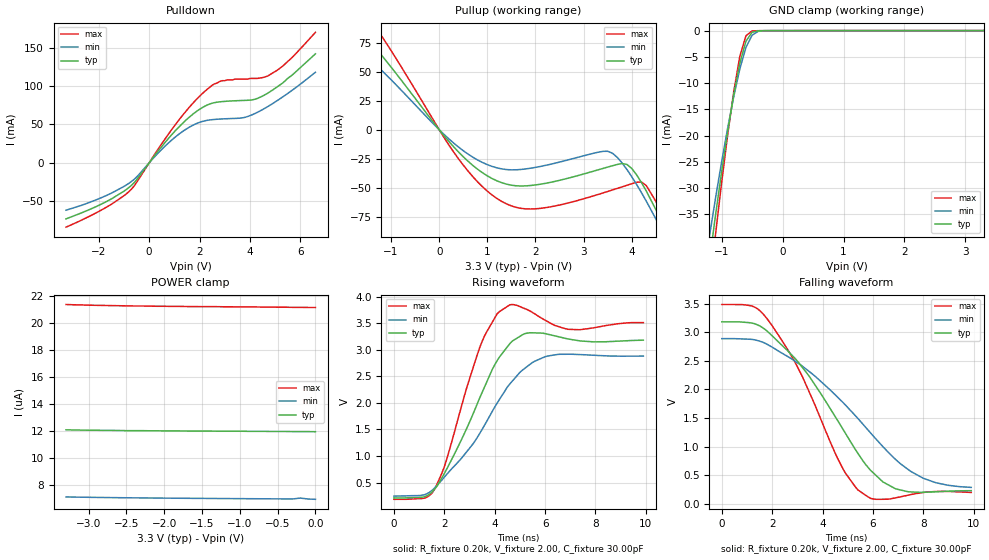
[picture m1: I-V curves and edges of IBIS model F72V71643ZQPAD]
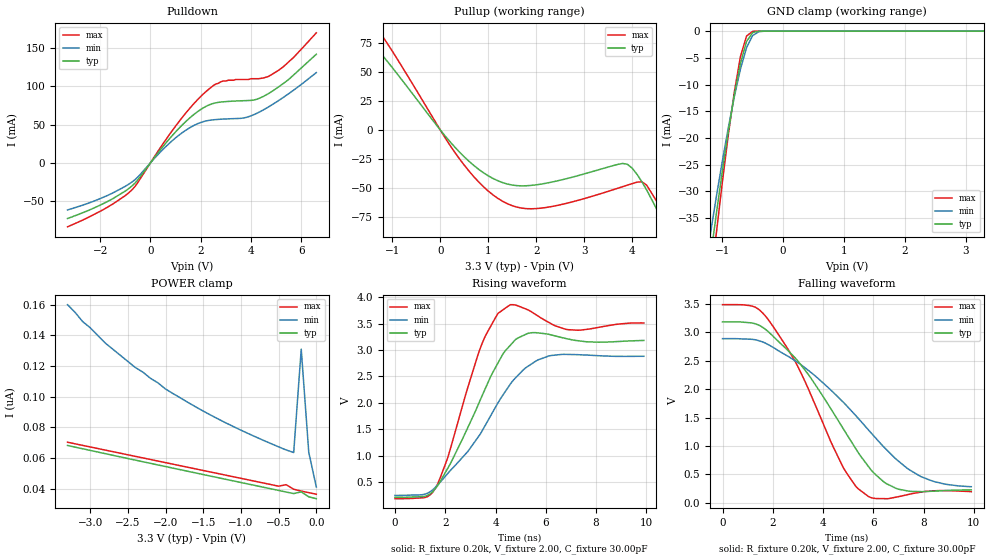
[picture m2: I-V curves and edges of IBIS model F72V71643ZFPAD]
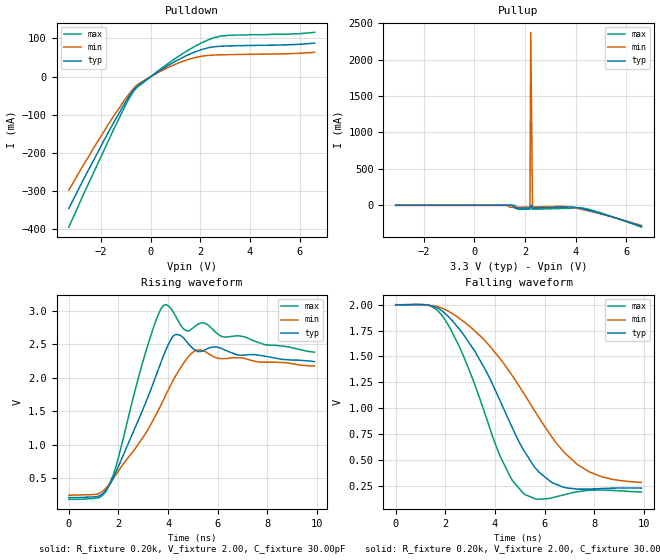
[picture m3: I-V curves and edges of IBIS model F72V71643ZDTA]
| IBIS file f72v7164.ibs created by s2ibis2 version 1.1
| North Carolina State University Electronics Research Laboratory  1995
[IBIS ver]   2.1
[File name]   f72v7164.ibs
[File Rev]   1.0
[Date]   09/11/2000
[Source]   Integrated Device Technology, Inc.
[Notes]   1. Temperatures: typ=25C, min=85C, max=-40C 2. Cemos9_3v
   process. 3. Ramp rates based on 50 ohm load.
[Copyright]   Copyright 1999, Integrated Device Technology, Inc.
|   Component idt72v71643z
[Component]   idt72v71643z
[Manufacturer]   Integrated Device Technology
[Package]
| variable   typ   min   max
R_pkg   0.75   0.60   0.90
L_pkg   8.10nH   8.30nH   9.90nH
C_pkg   0.53pF   0.46pF   0.60pF
[Pin]  signal_name   model_name   R_pin   L_pin   C_pin
1   ODE   F72V71643ZTTL
2   RESET   F72V71643ZTTL
3   GND   GND
4   CLK   F72V71643ZTTL
5   FOI   F72V71643ZTTL
6   FE_HCLK   F72V71643ZTTL
7   WFPS   F72V71643ZTTL
8   VCC   POWER
9   TMS   F72V71643ZTTLPU
10   TDI   F72V71643ZTTLPU
11   TDO   F72V71643ZFPAD
12   TCK   F72V71643ZTTL
13   TRST   F72V71643ZTTLPU
14   GND   GND
15   DS   F72V71643ZTTL
16   CS   F72V71643ZTTL
17   R_W   F72V71643ZTTL
18   VCC   POWER
19   A0   F72V71643ZTTL
20   A1   F72V71643ZTTL
21   A2   F72V71643ZTTL
22   A3   F72V71643ZTTL
23   A4   F72V71643ZTTL
24   A5   F72V71643ZTTL
25   GND   GND
26   A6   F72V71643ZTTL
27   A7   F72V71643ZTTL
28   A8   F72V71643ZTTL
29   A9   F72V71643ZTTL
30   A10   F72V71643ZTTL
31   A11   F72V71643ZTTL
32   A12   F72V71643ZTTL
33   A13   F72V71643ZTTL
34   A14   F72V71643ZTTL
35   DTA   F72V71643ZDTA
36   VCC   POWER
37   D15   F72V71643ZQPAD
38   D14   F72V71643ZQPAD
39   GND   GND
40   D13   F72V71643ZQPAD
41   D12   F72V71643ZQPAD
42   VCC   POWER
43   D11   F72V71643ZQPAD
44   D10   F72V71643ZQPAD
45   GND   GND
46   D9   F72V71643ZQPAD
47   D8   F72V71643ZQPAD
48   VCC   POWER
49   D7   F72V71643ZQPAD
50   D6   F72V71643ZQPAD
51   GND   GND
52   D5   F72V71643ZQPAD
53   D4   F72V71643ZQPAD
54   VCC   POWER
55   D3   F72V71643ZQPAD
56   D2   F72V71643ZQPAD
57   GND   GND
58   D1   F72V71643ZQPAD
59   D0   F72V71643ZQPAD
60   VCC   POWER
61   TX31   F72V71643ZFPAD
62   TX30   F72V71643ZFPAD
63   GND   GND
64   TX29   F72V71643ZFPAD
65   TX28   F72V71643ZFPAD
66   VCC   POWER
67   TX27   F72V71643ZFPAD
68   TX26   F72V71643ZFPAD
69   GND   GND
70   TX25   F72V71643ZFPAD
71   TX24   F72V71643ZFPAD
72   VCC   POWER
73   RX31   F72V71643ZTTL
74   RX30   F72V71643ZTTL
75   Rx29   F72V71643ZTTL
76   RX28   F72V71643ZTTL
77   RX27   F72V71643ZTTL
78   RX26   F72V71643ZTTL
79   RX25   F72V71643ZTTL
80   RX24   F72V71643ZTTL
81   GND   GND
82   TX23   F72V71643ZFPAD
83   TX22   F72V71643ZFPAD
84   VCC   POWER
85   TX21   F72V71643ZFPAD
86   TX20   F72V71643ZFPAD
87   GND   GND
88   TX19   F72V71643ZFPAD
89   TX18   F72V71643ZFPAD
90   VCC   POWER
91   TX17   F72V71643ZFPAD
92   TX16   F72V71643ZFPAD
93   GND   GND
94   RX23   F72V71643ZTTL
95   RX22   F72V71643ZTTL
96   RX21   F72V71643ZTTL
97   RX20   F72V71643ZTTL
98   RX19   F72V71643ZTTL
99   RX18   F72V71643ZTTL
100   RX17   F72V71643ZTTL
101   RX16   F72V71643ZTTL
102   VCC   POWER
103   TX15   F72V71643ZFPAD
104   TX14   F72V71643ZFPAD
105   GND   GND
106   TX13   F72V71643ZFPAD
107   TX12   F72V71643ZFPAD
108   VCC   POWER
109   TX11   F72V71643ZFPAD
110   TX10   F72V71643ZFPAD
111   GND   GND
112   TX9   F72V71643ZFPAD
113   TX8   F72V71643ZFPAD
114   VCC   POWER
115   RX15   F72V71643ZTTL
116   RX14   F72V71643ZTTL
117   RX13   F72V71643ZTTL
118   RX12   F72V71643ZTTL
119   RX11   F72V71643ZTTL
120   RX10   F72V71643ZTTL
121   RX9   F72V71643ZTTL
122   RX8   F72V71643ZTTL
123   GND   GND
124   TX7   F72V71643ZFPAD
125   TX6   F72V71643ZFPAD
126   VCC   POWER
127   TX5   F72V71643ZFPAD
128   TX4   F72V71643ZFPAD
129   GND   GND
130   TX3   F72V71643ZFPAD
131   TX2   F72V71643ZFPAD
132   VCC   POWER
133   TX1   F72V71643ZFPAD
134   TX0   F72V71643ZFPAD
135   GND   GND
136   RX7   F72V71643ZTTL
137   RX6   F72V71643ZTTL
138   RX5   F72V71643ZTTL
139   RX4   F72V71643ZTTL
140   RX3   F72V71643ZTTL
141   RX2   F72V71643ZTTL
142   RX1   F72V71643ZTTL
143   RX0   F72V71643ZTTL
144   VCC   POWER
| Models and submodels in the file (5): F72V71643ZQPAD (I/O), F72V71643ZFPAD (3-state), F72V71643ZDTA (Output), F72V71643ZTTL (Input), F72V71643ZTTLPU (Input)
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| FIN  FIN   dummy_model
| FOEL FOEL   dummy_model
| QIN  QIN   dummy_model
| QOEL QOEL   dummy_model
| DIN  DIN   dummy_model
|   Model F72V71643ZQPAD
[Model]   F72V71643ZQPAD
Model_type   I/O
Polarity   Non-Inverting
Enable   Active-Low
Vinl =  0.000V
Vinh =  3.000V
Vmeas =  1.500V
C_comp   3.00pF   NA   NA
[Temperature Range]   25.00   85.00   -40.00
[Voltage Range]   3.30V   3.00V   3.60V
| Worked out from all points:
|   slope of the pulldown table from 0 to 0.495 V, typ, clamps not added: 23.4 ohm
|   slope of the pullup table from 0 to 0.495 V, typ, clamps not added: 21.5 ohm
|   GND clamp passes 1 mA (typ) near -0.54 V on its own axis
|   rising waveform, R_fixture 0.20k, V_fixture 2.00, C_fixture 30.00pF: 20-80 % time 1.71ns typ, 2.27ns min, 1.23ns max; typ from 0.211 V to 3.18 V
|   falling waveform, R_fixture 0.20k, V_fixture 2.00, C_fixture 30.00pF: 20-80 % time 2.7ns typ, 3.51ns min, 2.11ns max; typ from 3.18 V to 0.229 V
[Pulldown]
| voltage   I(typ)   I(min)   I(max)
-3.3V     -72.9mA    -61.6mA    -83.7mA
-1.7V     -50.47mA   -42.52mA   -57.8mA
-800mV    -32mA      -26.54mA   -37.34mA
1.2V      47.36mA    37.84mA    56.62mA
1.9V      67.48mA    51.48mA    83.43mA
2.5V      77.68mA    56.27mA    101mA
2.9V      79.82mA    57.23mA    107mA
3.8V      81.37mA    59.31mA    109mA
4.2V      82.87mA    64.29mA    110mA
4.7V      90.61mA    73.16mA    113mA
5.3V      104mA      85.84mA    126mA
6.6V      142mA      118mA      170mA
[Pullup]
| voltage   I(typ)   I(min)   I(max)
-3.3V     146mA      42.93mA    190mA
-3.1V     142mA      104mA      183mA
-2.3V     116mA      90.89mA    147mA
-1.7V     89.49mA    71.08mA    113mA
-1V       53.97mA    43.08mA    68.23mA
400mV     -19.12mA   -14.86mA   -24.97mA
1.4V      -46.87mA   -34.3mA    -63.88mA
3.5V      -32.15mA   -18.55mA   -53.15mA
3.9V      -29.89mA   -34.29mA   -47.82mA
4.2V      -45.33mA   -54.06mA   -44.96mA
4.7V      -86.49mA   -93.01mA   -79.56mA
6.6V      -284mA     -270mA     -297mA
[GND_clamp]
| voltage   I(typ)   I(min)   I(max)
-3.3V     -263mA     -228mA     -298mA
-1.2V     -43.96mA   -39.28mA   -49.29mA
-1.1V     -35.25mA   -32mA      -38.93mA
-1V       -26.98mA   -25.08mA   -29.06mA
-900mV    -19.24mA   -18.57mA   -19.87mA
-800mV    -12.2mA    -12.56mA   -11.61mA
-700mV    -6.204mA   -7.29mA    -4.893mA
-600mV    -2.013mA   -3.2mA     -972uA
-500mV    -309uA     -878uA     -70.81uA
-400mV    -29.79uA   -143uA     -9.433uA
-300mV    -4.914uA   -18.95uA   -5.467uA
3.3V      11.96uA    6.997uA    21.11uA
[POWER_clamp]
| voltage   I(typ)   I(min)   I(max)
-3.3V     12.1uA     7.147uA    21.35uA
-3V       12.07uA    7.12uA     21.3uA
-2.4V     12.04uA    7.079uA    21.24uA
-2V       12.02uA    7.059uA    21.22uA
-1.5V     12.01uA    7.039uA    21.19uA
-1.3V     12uA       7.031uA    21.19uA
-800mV    11.99uA    7.014uA    21.17uA
-400mV    11.98uA    7uA        21.15uA
-300mV    11.97uA    6.997uA    21.14uA
-200mV    11.97uA    7.063uA    21.14uA
-100mV    11.97uA    6.994uA    21.13uA
0V        11.96uA    6.97uA     21.13uA
[Ramp]
| variable   typ   min   max
dV/dt_r   1.29/1.36n   1.01/2.24n   1.57/0.86n
dV/dt_f   1.28/3.06n   1.01/4.04n   1.50/2.19n
R_load = 50.00
[Rising Waveform]
R_fixture = 0.20k
V_fixture = 2.00
C_fixture = 30.00pF
R_dut = 0.75
L_dut = 8.10nH
C_dut = 0.53pF
| time   V(typ)   V(min)   V(max)
0s        211mV      247mV      185mV
1.2ns     232mV      271mV      206mV
1.6ns     370mV      392mV      364mV
2ns       670mV      602mV      797mV
3.4ns     2.089V     1.421V     3.037V
4.2ns     2.871V     2.074V     3.723V
5.1ns     3.283V     2.617V     3.794V
6ns       3.305V     2.87V      3.558V
7.3ns     3.174V     2.912V     3.379V
9.9ns     3.182V     2.882V     3.512V
[Falling Waveform]
R_fixture = 0.20k
V_fixture = 2.00
C_fixture = 30.00pF
R_dut = 0.75
L_dut = 8.10nH
C_dut = 0.53pF
| time   V(typ)   V(min)   V(max)
0s        3.18V      2.886V     3.483V
1.2ns     3.158V     2.873V     3.455V
1.9ns     2.977V     2.762V     3.172V
3.4ns     2.269V     2.335V     2.021V
4.6ns     1.452V     1.861V     789mV
5.4ns     881mV      1.491V     242mV
6ns       545mV      1.19V      84.65mV
6.9ns     261mV      773mV      104mV
8ns       201mV      445mV      197mV
9.9ns     229mV      286mV      198mV
|   Model F72V71643ZFPAD
[Model]   F72V71643ZFPAD
Model_type   3-state
Polarity   Non-Inverting
Enable   Active-Low
Vinl =  0.000V
Vinh =  3.000V
Vmeas =  1.500V
C_comp   3.00pF   NA   NA
[Temperature Range]   25.00   85.00   -40.00
[Voltage Range]   3.30V   3.00V   3.60V
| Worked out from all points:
|   slope of the pulldown table from 0 to 0.495 V, typ, clamps not added: 23.4 ohm
|   slope of the pullup table from 0 to 0.495 V, typ, clamps not added: 21.5 ohm
|   GND clamp passes 1 mA (typ) near -0.54 V on its own axis
|   rising waveform, R_fixture 0.20k, V_fixture 2.00, C_fixture 30.00pF: 20-80 % time 1.75ns typ, 2.28ns min, 1.25ns max; typ from 0.211 V to 3.18 V
|   falling waveform, R_fixture 0.20k, V_fixture 2.00, C_fixture 30.00pF: 20-80 % time 2.7ns typ, 3.51ns min, 2.12ns max; typ from 3.18 V to 0.229 V
[Pulldown]
| voltage   I(typ)   I(min)   I(max)
-3.3V     -72.8mA    -61.6mA    -83.7mA
-1.9V     -53.7mA    -45.35mA   -61.6mA
-800mV    -32.01mA   -26.54mA   -37.34mA
1.2V      47.36mA    37.84mA    56.62mA
1.9V      67.48mA    51.49mA    83.43mA
2.5V      77.68mA    56.27mA    101mA
2.9V      79.82mA    57.23mA    107mA
3.8V      81.36mA    59.3mA     109mA
4.2V      82.85mA    64.29mA    110mA
4.7V      90.6mA     73.15mA    113mA
5.3V      104mA      85.84mA    126mA
6.6V      142mA      118mA      170mA
[Pullup]
| voltage   I(typ)   I(min)   I(max)
-3.3V     146mA      NA         190mA
-1.7V     89.49mA    NA         113mA
-1.5V     79.73mA    NA         100mA
-1V       53.97mA    NA         68.23mA
400mV     -19.13mA   NA         -24.99mA
1.4V      -46.88mA   NA         -63.9mA
2.2V      -46.21mA   NA         -67.17mA
3.9V      -29.82mA   NA         -47.81mA
4.3V      -51.98mA   NA         -47.82mA
4.7V      -85.13mA   NA         -78.74mA
4.9V      -103mA     NA         -98.49mA
6.6V      -279mA     NA         -292mA
[GND_clamp]
| voltage   I(typ)   I(min)   I(max)
-3.3V     -257mA     -223mA     -293mA
-1.2V     -42.98mA   -38.32mA   -48.28mA
-1.1V     -34.44mA   -31.21mA   -38.11mA
-1V       -26.34mA   -24.44mA   -28.43mA
-900mV    -18.77mA   -18.08mA   -19.41mA
-800mV    -11.88mA   -12.22mA   -11.32mA
-700mV    -6.026mA   -7.079mA   -4.749mA
-600mV    -1.941mA   -3.095mA   -929uA
-500mV    -292uA     -843uA     -59.24uA
-400mV    -24.21uA   -135uA     -2.054uA
-300mV    -1.459uA   -16.11uA   -49.55nA
3.3V      33.5nA     63.6nA     33.36nA
[POWER_clamp]
| voltage   I(typ)   I(min)   I(max)
-3.3V     68.2nA     160nA      70.31nA
-3.1V     66.06nA    149nA      68.26nA
-2.8V     62.87nA    135nA      65.19nA
-2.4V     58.64nA    119nA      61.1nA
-2V       54.45nA    105nA      57nA
-1.2V     46.12nA    82.93nA    48.82nA
-500mV    38.89nA    67.3nA     41.66nA
-400mV    37.85nA    65.27nA    42.62nA
-300mV    36.82nA    63.6nA     39.66nA
-200mV    37.97nA    131nA      38.46nA
-100mV    34.71nA    63.7nA     37.43nA
0V        33.5nA     41.17nA    36.41nA
[Ramp]
| variable   typ   min   max
dV/dt_r   1.29/1.37n   1.01/2.24n   1.57/0.93n
dV/dt_f   1.28/3.05n   1.01/4.05n   1.50/2.17n
R_load = 50.00
[Rising Waveform]
R_fixture = 0.20k
V_fixture = 2.00
C_fixture = 30.00pF
R_dut = 0.75
L_dut = 8.10nH
C_dut = 0.53pF
| time   V(typ)   V(min)   V(max)
0s        211mV      247mV      185mV
1.6ns     375mV      396mV      377mV
2.1ns     762mV      664mV      964mV
3.5ns     2.172V     1.497V     3.165V
4.1ns     2.758V     2.003V     3.695V
4.5ns     3.045V     2.293V     3.831V
5.3ns     3.318V     2.696V     3.76V
6.2ns     3.289V     2.896V     3.502V
7.3ns     3.176V     2.912V     3.376V
9.9ns     3.182V     2.882V     3.513V
[Falling Waveform]
R_fixture = 0.20k
V_fixture = 2.00
C_fixture = 30.00pF
R_dut = 0.75
L_dut = 8.10nH
C_dut = 0.53pF
| time   V(typ)   V(min)   V(max)
0s        3.18V      2.886V     3.483V
1.2ns     3.158V     2.873V     3.455V
1.8ns     3.016V     2.786V     3.232V
3ns       2.492V     2.465V     2.394V
4.8ns     1.307V     1.772V     626mV
5.3ns     955mV      1.536V     294mV
5.8ns     644mV      1.286V     115mV
6.5ns     344mV      947mV      74.8mV
7.8ns     200mV      486mV      183mV
9.9ns     229mV      285mV      198mV
|   Model F72V71643ZDTA
[Model]   F72V71643ZDTA
Model_type   Output
Vmeas =  1.500V
C_comp   3.00pF   NA   NA
[Temperature Range]   25.00   85.00   -40.00
[Voltage Range]   3.30V   3.00V   3.60V
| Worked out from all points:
|   slope of the pulldown table from 0 to 0.495 V, typ, clamps not added: 23.4 ohm
|   rising waveform, R_fixture 0.20k, V_fixture 2.00, C_fixture 30.00pF: 20-80 % time 1.39ns typ, 1.93ns min, 904ps max; typ from 0.211 V to 2.24 V
|   falling waveform, R_fixture 0.20k, V_fixture 2.00, C_fixture 30.00pF: 20-80 % time 2.27ns typ, 3.02ns min, 1.71ns max; typ from 2 V to 0.227 V
[Pulldown]
| voltage   I(typ)   I(min)   I(max)
-3.3V     -345mA     -297mA     -394mA
-1.7V     -145mA     -124mA     -167mA
-1V       -64.57mA   -56.38mA   -72.75mA
-700mV    -35.55mA   -31.63mA   -39.13mA
-500mV    -22.44mA   -19.4mA    -25.6mA
400mV     17.24mA    14.26mA    20.09mA
1.2V      47.36mA    37.84mA    56.62mA
2V        69.73mA    52.76mA    86.75mA
2.6V      78.47mA    56.58mA    103mA
3.4V      80.84mA    57.89mA    109mA
5.5V      83.3mA     59.95mA    111mA
6.6V      87.77mA    63.64mA    116mA
[Pullup]
| voltage   I(typ)   I(min)   I(max)
-3.1V     66.07nA    150nA      68.27nA
1.3V      20.24nA    25.11nA    23.2nA
1.5V      18.19nA    -27.64mA   21.15nA
1.6V      -38.62mA   -27.6mA    20.12nA
1.7V      -38.76mA   -27.36mA   -54.17mA
2.2V      -36.97mA   -24.61mA   -53.74mA
2.23V     68.2nA     2.374A     70.31nA
2.3V      -36.31mA   -23.87mA   -53.19mA
3.5V      -25.71mA   -15.02mA   -42.52mA
4.3V      -48.22mA   -59.72mA   -39.45mA
5.1V      -123mA     -128mA     -116mA
6.6V      -289mA     -277mA     -300mA
[Ramp]
| variable   typ   min   max
dV/dt_r   1.11/1.39n   0.83/2.31n   1.38/0.89n
dV/dt_f   1.28/3.04n   1.01/4.06n   1.51/2.20n
R_load = 50.00
[Rising Waveform]
R_fixture = 0.20k
V_fixture = 2.00
C_fixture = 30.00pF
R_dut = 0.75
L_dut = 8.10nH
C_dut = 0.53pF
| time   V(typ)   V(min)   V(max)
0s        211mV      247mV      185mV
1.5ns     321mV      352mV      307mV
1.9ns     591mV      554mV      672mV
3.1ns     1.631V     1.17V      2.385V
3.8ns     2.312V     1.659V     3.07V
4.3ns     2.642V     2.024V     2.919V
4.7ns     2.557V     2.255V     2.706V
5.2ns     2.387V     2.413V     2.795V
6.2ns     2.425V     2.283V     2.609V
9.9ns     2.238V     2.174V     2.379V
[Falling Waveform]
R_fixture = 0.20k
V_fixture = 2.00
C_fixture = 30.00pF
R_dut = 0.75
L_dut = 8.10nH
C_dut = 0.53pF
| time   V(typ)   V(min)   V(max)
0s        2V         2V         2V
1.3ns     1.996V     1.997V     1.997V
1.9ns     1.934V     1.963V     1.885V
2.8ns     1.687V     1.825V     1.463V
4.2ns     1.075V     1.48V      540mV
5.2ns     578mV      1.128V     166mV
6.3ns     280mV      719mV      134mV
7.3ns     218mV      459mV      191mV
8.3ns     223mV      337mV      209mV
9.9ns     227mV      283mV      190mV
